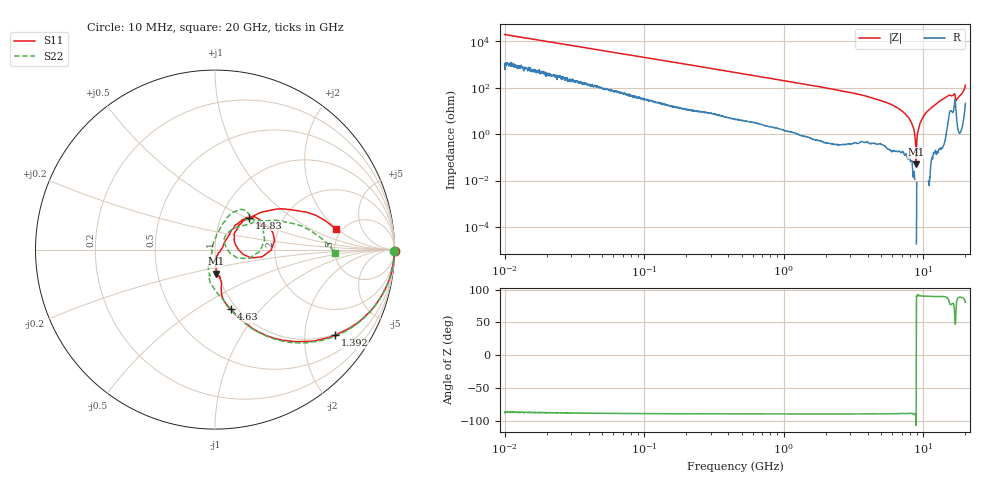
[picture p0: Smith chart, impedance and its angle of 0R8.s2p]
!Keysight Technologies,P5008B,MY61100088,A.16.20.02
!Date: Friday, August 30, 2024 10:43:57
!Correction: S11(C  2-Port  )
!S21(C  2-Port  )
!S12(C  2-Port  )
!S22(C  2-Port  )
!S2P File: Measurements: S11, S21, S12, S22:Log Frequency Sweep
# Hz S  dB  R 50
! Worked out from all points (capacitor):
!   1601 points, 10 MHz to 20 GHz, reference 50 ohm
!   read as one part in series: C = 821 fF near 10.39 MHz
!   lowest |Z| = 50.5 mohm at 8.876 GHz (marker M1)
!   series resonance near 8.885 GHz, so ESL is about 390 pH
!   S11 on the Smith chart (normalised r, x): 10 MHz: open; 1.392 GHz: 0.96, -2.82; 4.63 GHz: 0.93, -0.71; 14.83 GHz: 1.36, +0.52; 20 GHz: 4.47, +1.91
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1e7  0.00 -0.3  -45.75 86.7  -45.76 87.2  -0.00 -0.3
3.555162e7  -0.01 -1.1  -34.88 87.2  -34.88 87.2  -0.01 -1.1
1.263918e8  -0.03 -3.7  -24.05 85.5  -24.05 85.5  -0.02 -3.8
4.472136e8  -0.23 -12.8  -13.35 76.5  -13.35 76.5  -0.22 -13.0
8.137127e8  -0.67 -22.5  -8.61 66.9  -8.61 66.9  -0.67 -22.8
1.391895e9  -1.71 -35.6  -4.94 53.8  -4.94 53.8  -1.71 -36.2
1.589917e9  -2.14 -39.6  -4.15 49.8  -4.16 49.8  -2.14 -40.3
2.681144e9  -4.62 -56.7  -1.87 32.8  -1.87 32.7  -4.61 -57.2
4.630008e9  -9.26 -75.3  -0.57 14.1  -0.57 14.1  -9.26 -75.1
5.652411e9  -11.28 -81.2  -0.34 7.4  -0.34 7.3  -11.36 -82.7
8.876309e9  -17.43 -87.6  -0.05 -7.5  -0.05 -7.6  -17.54 -104.9
1.033363e10  -22.45 -86.9  0.02 -13.0  0.01 -13.1  -22.48 -113.3
1.130974e10  -29.14 -67.5  0.04 -16.6  0.03 -16.7  -30.38 -130.2
1.169216e10  -30.62 -31.8  0.03 -18.1  0.03 -18.2  -34.78 -177.2
1.197321e10  -29.52 1.1  0.03 -19.1  0.03 -19.2  -33.36 128.5
1.316659e10  -17.55 48.7  -0.03 -24.2  -0.03 -24.3  -17.90 75.5
1.482695e10  -11.68 43.1  -0.37 -33.3  -0.37 -33.4  -11.90 59.8
1.630478e10  -10.86 29.5  -0.97 -36.2  -0.97 -36.3  -11.89 42.4
1.693636e10  -11.52 -8.7  -2.10 -28.0  -2.10 -28.1  -14.12 -14.4
1.767617e10  -17.08 40.0  -0.19 -35.7  -0.19 -35.9  -18.07 52.0
1.871311e10  -11.61 42.7  -0.40 -47.1  -0.40 -47.3  -11.73 35.4
2e10  -3.30 9.6  -4.18 -74.1  -4.18 -74.3  -3.47 -1.8
